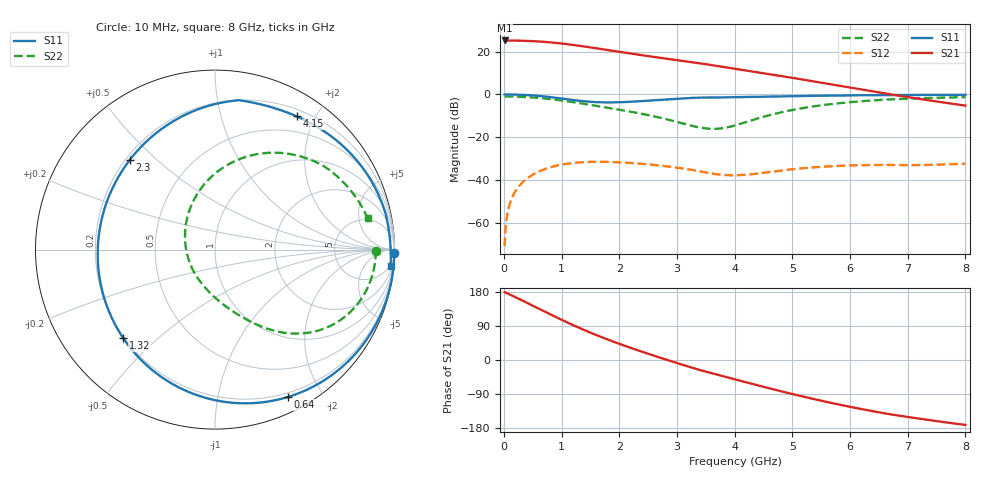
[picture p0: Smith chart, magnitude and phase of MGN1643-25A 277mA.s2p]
! Port[1] = GATE
! Port[2] = DRAIN
! [Type]  S-parameter s2p file touchstone ver. 1.0
! [Object]  MGN1643-25A
! [Bias]  277 mA
! [Version]  1.0
! [Date]  Tue May 19 13:03:48 2026
! [Source]  This file was created in JSC "ICC Milandr".
! [Disclaimer] Property of JSC "ICC Milandr". Unauthorized reproduction and/or distribution is strictly prohibited.
!  The file and the data are provided "AS IS" and with all faults and disclaim all warranties, express and implied, including
!  without limitation any implied warranties of merchantability, fitness for a particular purpose.
!  JSC "ICC Milandr" assumes no liability for:
!  1) the accuracy of the data provided;
!  2) the proper functioning of this data;
!  3) infringement of patents, copyrights or intellectual property rights resulting from the use of this data.
!  JSC "ICC Milandr" reserves the right to make changes to the products and the data without prior notice.
!  Please, be aware that your receipt and use of the file provided shall serve as acceptance of these terms and conditions.
!  If you do not accept these terms, you should return or destroy this file and any other accompanying information immediately.
# Hz S MA R 12.5
! freq  S11mag  S11ang  S21mag  S21ang  S12mag  S12ang  S22mag  S22ang
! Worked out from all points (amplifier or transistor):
!   800 points, 10 MHz to 8 GHz, reference 12.5 ohm
!   highest |S21| = 25.3 dB at 10 MHz (marker M1)
!   |S21| within 3 dB of that: start of sweep to 1.435 GHz
!   unconditionally stable (mu >= 1): 2.1 GHz to 6.021 GHz
!   at 1.34 GHz: K = 0.58, MSG = 27.2 dB, |S12| = -31.7 dB
!   at 4.01 GHz: K = 2.27, MAG = 18.6 dB, |S12| = -37.8 dB
!   at 8 GHz: K = 0.45, MSG = 13.6 dB, |S12| = -32.4 dB
!   S11 on the Smith chart (normalised r, x): 10 MHz: open; 640 MHz: 0.16, -1.60; 1.32 GHz: 0.20, -0.39; 2.3 GHz: 0.22, +0.41; 4.15 GHz: 0.28, +1.75; 8 GHz: 4, -21
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1e7  0.9997 -0.9  18.4 179.1  0.0002816 81.7  0.8958 -0.4
1.1e8  0.9982 -10.7  18.32 172.1  0.00305 82.4  0.8944 -4.5
3.2e8  0.9815 -31.3  18.11 156.7  0.008754 69.4  0.8793 -13.1
4.7e8  0.9569 -46.2  17.81 145.5  0.0126 59.7  0.8581 -19.1
6.4e8  0.9164 -63.6  17.29 132.6  0.01655 48.5  0.8239 -25.8
8e8  0.8688 -80.2  16.63 120.6  0.01973 38.1  0.7833 -31.8
9.6e8  0.8167 -97.2  15.82 108.8  0.0223 28.0  0.7369 -37.4
1.13e9  0.7623 -115.5  14.86 96.7  0.02432 17.6  0.6842 -42.9
1.32e9  0.7104 -136.0  13.72 83.7  0.02577 6.7  0.625 -48.3
1.35e9  0.7035 -139.2  13.54 81.7  0.02592 5.0  0.6158 -49.1
1.57e9  0.666 -162.5  12.24 67.7  0.02656 -6.5  0.5509 -54.6
1.79e9  0.6523 175.7  11.02 54.5  0.02646 -17.2  0.4915 -59.7
2.03e9  0.6605 154.2  9.829 41.0  0.02573 -27.7  0.4326 -65.2
2.3e9  0.6892 133.6  8.663 26.6  0.02439 -38.6  0.3718 -72.1
2.68e9  0.7454 110.3  7.305 7.4  0.02188 -52.4  0.2917 -84.7
3.32e9  0.8404 81.6  5.58 -23.2  0.01664 -71.7  0.1767 -128.3
4.01e9  0.864 61.9  4.006 -51.4  0.01286 -53.3  0.1895 151.7
4.15e9  0.8708 58.5  3.746 -57.0  0.0131 -48.8  0.2162 138.4
4.74e9  0.9015 45.4  2.802 -80.1  0.01616 -40.0  0.365 100.0
5.34e9  0.9298 33.7  2.058 -102.0  0.01958 -43.6  0.5207 75.1
6.67e9  0.9712 12.1  1.026 -142.6  0.0225 -60.9  0.7651 37.3
8e9  0.9822 -5.3  0.5496 -171.4  0.02396 -84.2  0.868 11.7
